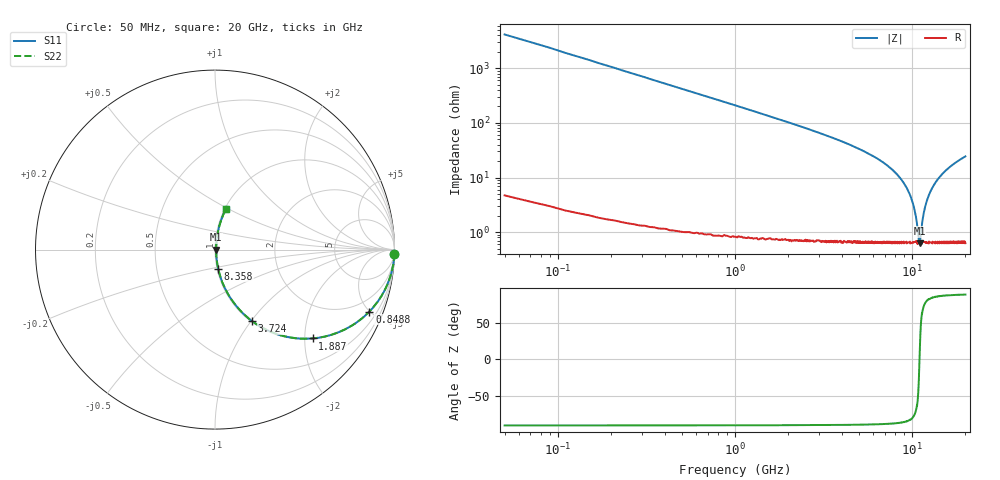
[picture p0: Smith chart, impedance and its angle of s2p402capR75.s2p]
! AVX Thin Film Operation		Date: September 2011
! Description: Accu-P® Series, Thin Film, SMD, RF Capacitor
! Part Number: 04021JR75ZBW/STR
! 50 MHz  -  20 GHz
! Serial Measurements
# MHZ S MA R 50
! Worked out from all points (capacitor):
!   1000 points, 50 MHz to 20 GHz, reference 50 ohm
!   read as one part in series: C = 749 fF near 149.8 MHz
!   lowest |Z| = 625 mohm at 11.01 GHz (marker M1)
!   series resonance near 11.01 GHz, so ESL is about 280 pH
!   S11 on the Smith chart (normalised r, x): 50 MHz: -0, -85; 848.8 MHz: 1.01, -4.97; 1.887 GHz: 1.01, -2.18; 3.724 GHz: 1.01, -1.01; 8.358 GHz: 1.01, -0.22; 20 GHz: 1.01, +0.49
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50  1 -1.4  0.024 88.6  0.024 88.6  1 -1.4
209.76  0.995 -5.6  0.098 84.3  0.098 84.3  0.995 -5.6
329.58  0.988 -8.8  0.154 81.1  0.154 81.1  0.988 -8.8
549.249  0.967 -14.5  0.251 75.3  0.251 75.3  0.967 -14.5
848.799  0.927 -21.9  0.373 67.9  0.373 67.9  0.927 -21.9
1887.237  0.735 -42.3  0.673 47.3  0.673 47.3  0.735 -42.3
3384.985  0.491 -59.9  0.865 29.4  0.865 29.4  0.491 -59.9
3724.474  0.448 -62.6  0.888 26.6  0.888 26.6  0.448 -62.6
6700  0.195 -76.9  0.975 11.2  0.975 11.2  0.195 -76.9
8357.508  0.107 -80.5  0.988 6.1  0.988 6.1  0.107 -80.5
9296.096  0.065 -80.6  0.991 3.7  0.991 3.7  0.065 -80.6
10034.99  0.036 -77.7  0.993 2.0  0.993 2.0  0.036 -77.7
10474.32  0.02 -70.4  0.993 1.1  0.993 1.1  0.02 -70.4
10893.69  0.007653 -32.7  0.994 0.2  0.994 0.2  0.007653 -32.7
11013.51  0.00642 0.2  0.994 -0.0  0.994 -0.0  0.00642 0.2
11113.36  0.007302 28.3  0.994 -0.2  0.994 -0.2  0.007302 28.3
11532.73  0.019 69.0  0.993 -1.0  0.993 -1.0  0.019 69.0
11912.16  0.031 76.2  0.993 -1.7  0.993 -1.7  0.031 76.2
12491.29  0.049 79.7  0.992 -2.8  0.992 -2.8  0.049 79.7
13350  0.074 80.8  0.991 -4.2  0.991 -4.2  0.074 80.8
16684.99  0.162 78.4  0.98 -9.3  0.98 -9.3  0.162 78.4
20000  0.236 74.8  0.966 -13.6  0.966 -13.6  0.236 74.8
